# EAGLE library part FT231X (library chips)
USB Bridge, USB to UART USB 2.0 UART Interface
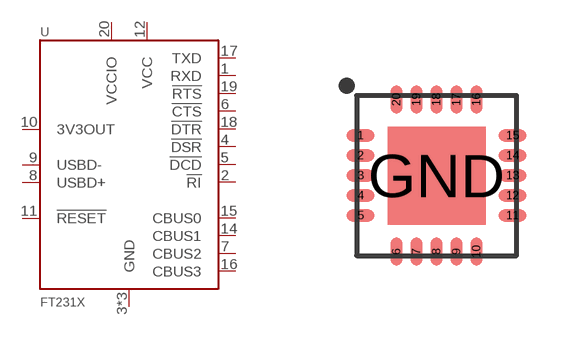
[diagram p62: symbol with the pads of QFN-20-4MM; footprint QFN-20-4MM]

Designator prefix U

## FT231XQ (DIGIKEY: 768-1128-1-ND; MPN: FT231XQ-R)  [QFN-20-4MM]
1  RXD
2  !RI
3  GND
4  !DSR
5  !DCD
6  !CTS
7  CBUS2
8  USBD+
9  USBD-
10  3V3OUT
11  !RESET
12  VCC
13  GND
14  CBUS1
15  CBUS0
16  CBUS3
17  TXD
18  !DTR
19  !RTS
20  VCCIO
GND  GND

## Footprint QFN-20-4MM (pad centres in mm)
smd 0.7 x 0.3: 1 -1.9,1; 2 -1.9,0.5; 3 -1.9,0; 4 -1.9,-0.5; 5 -1.9,-1; 11 1.9,-1; 12 1.9,-0.5; 13 1.9,0; 14 1.9,0.5; 15 1.9,1
smd 0.3 x 0.7: 6 -1,-1.9; 7 -0.5,-1.9; 8 0,-1.9; 9 0.5,-1.9; 10 1,-1.9; 16 1,1.9; 17 0.5,1.9; 18 0,1.9; 19 -0.5,1.9; 20 -1,1.9
smd 2.45 x 2.45: GND 0,0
